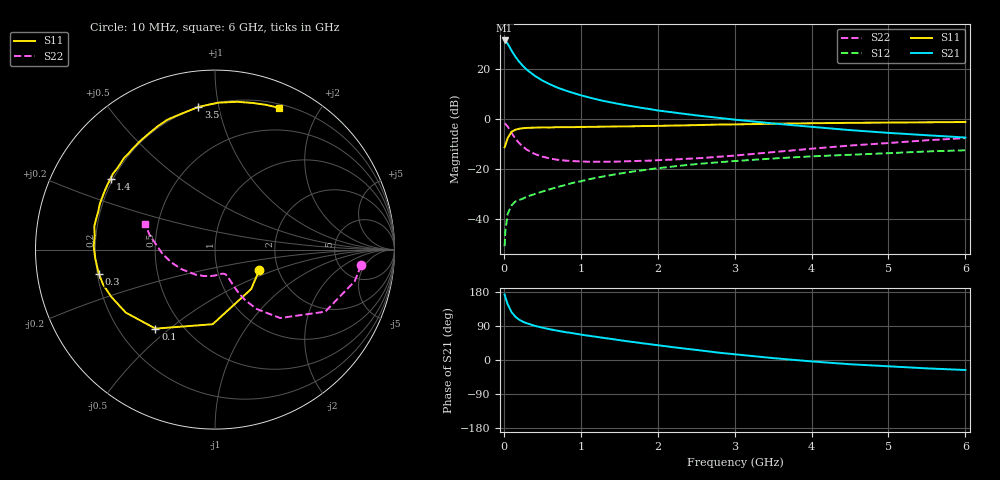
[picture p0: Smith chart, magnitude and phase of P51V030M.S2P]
! SIEMENS Small Signal Semiconductors
! BFP183
! Si NPN RF Bipolar Junction Transistor in SOT143
! VCE = 1 V  IC = 30 mA
! Common Emitter S-Parameters:  March  1996
# GHz  S  MA  R  50
!  f  S11  S21  S12  S22
! GHz  MAG  ANG  MAG  ANG  MAG  ANG  MAG  ANG
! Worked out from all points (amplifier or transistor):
!   36 points, 10 MHz to 6 GHz, reference 50 ohm
!   highest |S21| = 31.3 dB at 10 MHz (marker M1)
!   |S21| within 3 dB of that: start of sweep to 81.44 MHz
!   unconditionally stable (mu >= 1): start of sweep to 15.03 MHz; 321.4 MHz to end of sweep
!   at 250 MHz: K = 0.88, MSG = 26.4 dB, |S12| = -31.8 dB
!   at 1.4 GHz: K = 1.55, MAG = 10.1 dB, |S12| = -22.4 dB
!   at 6 GHz: K = 1.25, MAG = -0.5 dB, |S12| = -12.5 dB
!   S11 on the Smith chart (normalised r, x): 10 MHz: 1.59, -0.40; 100 MHz: 0.35, -0.45; 300 MHz: 0.21, -0.10; 1.4 GHz: 0.19, +0.30; 3.5 GHz: 0.20, +0.87; 6 GHz: 0.24, +1.52
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0.01  0.2717 -25.1  36.6 172.8  0.0029 77.7  0.8186 -6.2
0.02  0.2983 -47.5  36.05 165.8  0.0058 77.4  0.7978 -12.8
0.05  0.416 -91.8  31.55 147.0  0.0128 64.1  0.7046 -29.4
0.1  0.5513 -127.0  23.06 126.4  0.0189 49.2  0.5262 -46.4
0.15  0.6086 -144.8  17.38 114.2  0.0226 43.5  0.4036 -55.0
0.2  0.6349 -155.5  13.75 106.4  0.0241 43.0  0.3281 -59.1
0.25  0.6531 -162.7  11.26 100.8  0.0258 43.4  0.2781 -61.3
0.3  0.6613 -168.0  9.518 96.9  0.0283 44.8  0.2422 -62.4
0.4  0.6687 -175.6  7.267 90.3  0.0317 47.1  0.2004 -63.6
0.5  0.6762 178.5  5.817 85.4  0.0355 49.6  0.1769 -64.4
0.6  0.6746 173.5  4.892 81.0  0.0397 52.0  0.1623 -65.4
0.7  0.6848 169.2  4.178 77.2  0.0438 53.6  0.1526 -66.4
0.8  0.684 165.5  3.683 73.6  0.0482 54.2  0.1474 -67.8
1.1  0.6925 155.0  2.694 64.0  0.0623 55.3  0.1401 -73.8
1.4  0.703 145.9  2.121 55.6  0.0761 54.7  0.1401 -81.8
1.8  0.7194 134.8  1.652 44.2  0.0944 52.3  0.1457 -93.5
2.2  0.7351 124.4  1.346 33.8  0.1124 48.7  0.1544 -107.3
2.8  0.7707 110.2  1.045 19.2  0.1368 42.5  0.1764 -127.8
3.5  0.8004 96.6  0.811 5.0  0.1624 35.7  0.2172 -150.2
4.5  0.8332 81.3  0.597 -11.2  0.1927 25.4  0.2939 -175.4
5.5  0.8551 70.6  0.472 -22.1  0.2244 16.4  0.3745 167.2
6  0.8662 65.8  0.425 -26.4  0.2367 11.4  0.4144 159.8
